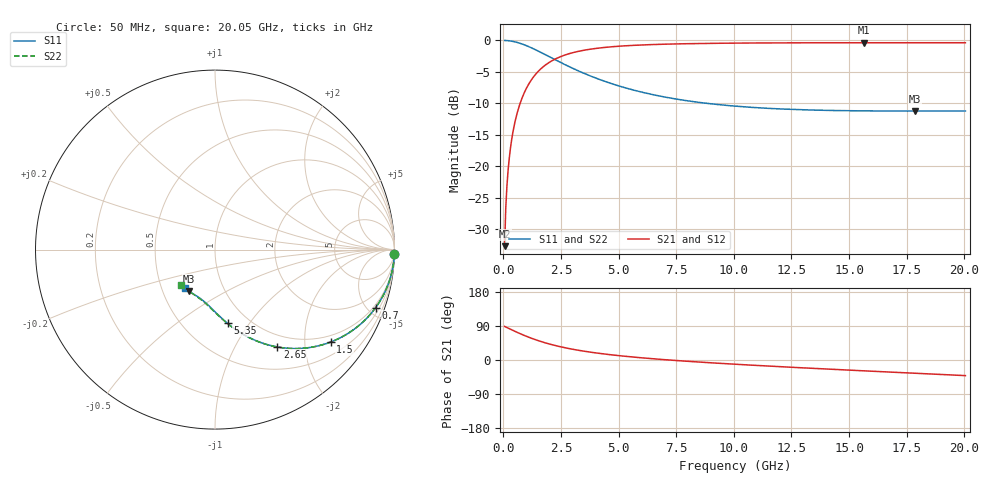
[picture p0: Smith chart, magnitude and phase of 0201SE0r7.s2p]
! AVX Thin Film Operation		Date: August 2001
! Description: Accu-P® Series, Thin Film, SMD, RF Capacitor
! Part Number: 02013J0R7ABW
! 50 MHz  -  20.05 GHz
! Serial Measurements
# mhz S db R 50
!	S11		S21		S12		S22
!	dB	Phase	dB	Phase	dB	Phase	dB	Phase
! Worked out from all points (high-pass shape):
!   401 points, 50 MHz to 20.05 GHz, reference 50 ohm
!   highest |S21| = -0.36 dB at 15.65 GHz (marker M1); lowest = -32.7 dB at 50 MHz (marker M2)
!   |S21| within 3 dB of the highest: 2.044 GHz to end of sweep
!   lowest |S11| = -11.2 dB at 17.85 GHz (marker M3), VSWR 1.76, Z = 33.8 - j16.9 ohm
!   |S11| at or under -10 dB: 8.807 GHz to end of sweep
!   |S22| runs from -11.3 to 0.0 dB; largest |S21 - S12| = 0
!   S11 on the Smith chart (normalised r, x): 50 MHz: 1, -78; 700 MHz: 0.82, -5.60; 1.5 GHz: 0.82, -2.63; 2.65 GHz: 0.81, -1.51; 5.35 GHz: 0.80, -0.79; 20.05 GHz: 0.65, -0.31
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50  -0.00 -1.5  -32.74 88.5  -32.74 88.5  -0.00 -1.5
100  -0.01 -2.9  -26.72 87.1  -26.72 87.1  -0.01 -2.9
200  -0.04 -5.8  -20.73 84.2  -20.73 84.2  -0.04 -5.8
250  -0.06 -7.3  -18.81 82.7  -18.81 82.7  -0.06 -7.3
300  -0.08 -8.7  -17.26 81.3  -17.26 81.3  -0.08 -8.7
450  -0.18 -13.0  -13.84 77.0  -13.84 77.0  -0.18 -13.0
550  -0.27 -15.8  -12.19 74.2  -12.19 74.2  -0.27 -15.8
700  -0.43 -19.9  -10.26 70.1  -10.26 70.1  -0.43 -19.9
1050  -0.91 -28.7  -7.24 61.2  -7.24 61.2  -0.91 -28.7
1500  -1.68 -38.7  -4.96 51.3  -4.96 51.3  -1.68 -38.7
2000  -2.61 -47.9  -3.46 42.1  -3.46 42.1  -2.61 -47.9
2650  -3.81 -57.3  -2.34 32.6  -2.34 32.6  -3.81 -57.4
3400  -5.08 -65.7  -1.62 24.2  -1.62 24.2  -5.08 -65.8
4300  -6.38 -73.4  -1.15 16.4  -1.15 16.4  -6.38 -73.5
5350  -7.61 -80.3  -0.84 9.4  -0.84 9.4  -7.61 -80.6
6750  -8.83 -87.5  -0.62 2.0  -0.62 2.0  -8.83 -88.0
10050  -10.45 -100.1  -0.43 -11.2  -0.43 -11.2  -10.47 -101.5
13400  -11.08 -110.3  -0.37 -21.9  -0.37 -21.9  -11.10 -112.8
15650  -11.21 -116.5  -0.36 -28.6  -0.36 -28.6  -11.24 -119.9
16750  -11.23 -119.4  -0.36 -31.8  -0.36 -31.8  -11.27 -123.3
17850  -11.24 -122.3  -0.36 -34.9  -0.36 -34.9  -11.28 -126.6
20050  -11.23 -128.0  -0.37 -41.2  -0.37 -41.2  -11.28 -133.3
